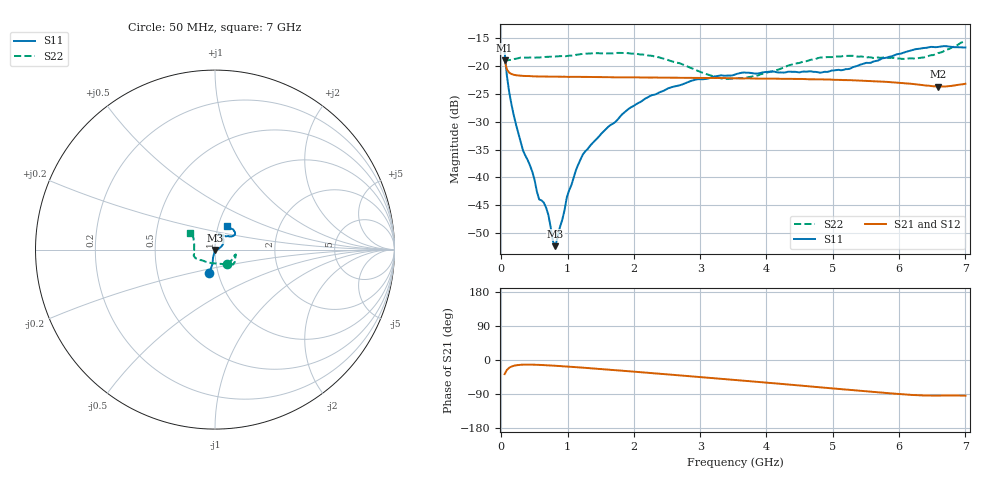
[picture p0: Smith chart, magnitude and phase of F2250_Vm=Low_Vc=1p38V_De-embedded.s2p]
! Integrated Device Technology
! Corporate Headquarters
! 6024 Silver Creek Valley Road
! San Jose, CA 95138  USA
! Phone:  1-408-284-8200
! Toll Free:  1-800-223-1366
! Webpage:  http://www.idt.com/
! Timing and RF Division
! 515 Groton Road, Suite 102
! Westford, MA 01886-6024
! Device:  F2250
! Description: Voltage Variable RF Attenuator
! Frequency:  50.0 -  6000.00 MHz
! Package:  3x3 mm Thin QFN Plastic Package: 16 pin
! Ports:  2 RF, 3 DC
!  Pin  1  = GND
!  Pin  2  = NC
!  Pin  3  = RF1  = Port 1
!  Pin  4  = NC
!  Pin  5  = GND
!  Pin  6  = GND
!  Pin  7  = GND
!  Pin  8  = GND
!  Pin  9  = NC
!  Pin 10  = RF2  = Port 2
!  Pin 11  = NC
!  Pin 12  = GND
!  Pin 13  = GND
!  Pin 14  = VCNTRL
!  Pin 15  = VDD
!  Pin 16  = VMODE
! Vcntrl:  1.380 Volts
! Vmode:  +0.000 Volts
! Vdd:  +3.30  Volts
! Current:  1.191 mA
! Data:  The device was measured on a the F2250 evaluation board which has
!  individual transmission lines to the RF pins.  Data was collected
!  using a calibrated network analyzer.  The evaluation board was
!  de-embedded using a TRL calibration technique.
!  The reference plane is the edge of the package pin.
! Misc:  SN 10
!  Action Tracker AT0258
! Date Measured:  2014-11-26
! Date:  2015-10-15  MJV
! Note:
!  Integrated Device Technology supplies this data as a sample of measured
!  data at the package pin for this product.  Your particular data for this
!  product may vary.
!  Data was taken at 25 degrees C.
!  Integrated Device Technology reserves the right to change this data at anytime.
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# GHz S dB R 50
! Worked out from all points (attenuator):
!   201 points, 50 MHz to 7 GHz, reference 50 ohm
!   highest |S21| = -18.95 dB at 50 MHz (marker M1); lowest = -23.7 dB at 6.583 GHz (marker M2)
!   lowest |S11| = -52.3 dB at 814.5 MHz (marker M3), VSWR 1.00, Z = 50.2 - j0.177 ohm
!   |S11| at or under -10 dB: start of sweep to end of sweep
!   |S22| runs from -22.3 to -15.4 dB; largest |S21 - S12| = 0.00027
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0.05  -17.46 -103.7  -18.95 -37.3  -18.94 -37.3  -19.36 -50.4
0.08475  -21.79 -99.9  -20.62 -26.3  -20.61 -26.3  -18.97 -26.5
0.1195  -24.71 -101.6  -21.18 -20.5  -21.18 -20.5  -18.93 -18.9
0.22375  -30.58 -103.4  -21.66 -13.9  -21.64 -13.9  -18.69 -14.2
0.328  -35.18 -104.4  -21.77 -12.3  -21.77 -12.3  -18.48 -13.4
0.467  -38.94 -108.4  -21.84 -12.3  -21.84 -12.3  -18.50 -14.5
0.57125  -43.95 -102.1  -21.88 -12.9  -21.86 -12.9  -18.47 -16.9
0.6755  -45.40 -86.6  -21.89 -13.8  -21.88 -13.8  -18.36 -19.1
0.71025  -46.73 -81.8  -21.90 -14.1  -21.88 -14.1  -18.34 -20.0
0.77975  -51.50 -63.8  -21.92 -14.8  -21.89 -14.8  -18.33 -21.5
0.8145  -52.34 -46.9  -21.91 -15.2  -21.91 -15.2  -18.30 -22.4
0.98825  -43.58 -18.6  -21.94 -17.2  -21.96 -17.2  -18.21 -26.1
1.2315  -35.86 6.6  -21.96 -20.2  -21.96 -20.2  -17.81 -30.5
1.9265  -27.63 27.3  -22.03 -29.8  -22.03 -29.8  -17.72 -39.3
2.37825  -24.76 37.1  -22.08 -36.1  -22.08 -36.1  -18.44 -45.7
2.93425  -22.44 52.8  -22.14 -44.1  -22.16 -44.1  -20.70 -61.2
3.525  -21.52 67.7  -22.21 -52.8  -22.21 -52.8  -22.22 -100.0
4.7065  -21.05 69.9  -22.37 -70.5  -22.40 -70.4  -18.84 -154.3
5.22775  -20.55 53.4  -22.52 -78.5  -22.54 -78.4  -18.18 -162.8
5.85325  -18.34 37.9  -22.88 -87.7  -22.88 -87.8  -18.54 -174.6
6.583  -16.59 44.1  -23.69 -94.0  -23.66 -94.1  -17.68 155.8
7  -16.67 62.7  -23.18 -94.1  -23.16 -94.3  -15.41 146.5
